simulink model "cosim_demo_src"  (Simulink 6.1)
settings: Solver=ode45  StartTime=0.0  StopTime=300  RelTol=1e-3
undefined symbols (not defined in the file or in its folder): netlist
libraries: xbsIndex_r3 x8

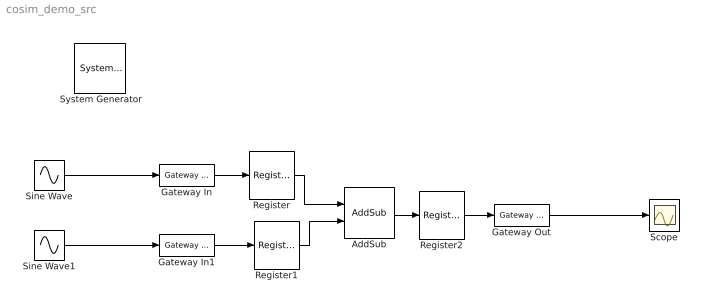
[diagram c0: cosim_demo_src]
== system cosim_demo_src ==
  " System Generator" : xbsIndex_r3/ System Generator  Tag=genX  xilinxfamily=Virtex2P  part=xc2vp70  speed=-5  package=ff1704  synthesis_tool=XST  directory=./netlist  testbench=off  simulink_period=1  sysclk_period=25  incr_netlist=off  trim_vbits=Everywhere in SubSystem  dbl_ovrd=According to Block Masks  core_generation=According to Block Masks  run_coregen=off  deprecated_control=off  eval_field=0
  AddSub : xbsIndex_r3/AddSub  mode=Addition  precision=Full  arith_type=Unsigned  n_bits=8  bin_pt=2  quantization=Truncate  overflow=Wrap  latency=0  explicit_period=off  period=1  use_carryin=off  use_carryout=off  en=off  dbl_ovrd=off  show_param=off  use_core=on  pipeline=off  use_rpm=off  gen_core=off
  Gateway In : xbsIndex_r3/Gateway In  arith_type="Signed  (2's comp)"  n_bits=12  bin_pt=0  quantization=Truncate  overflow=Wrap  period=1  timing_constraint=None  locs_specified=off  LOCs={}  needs_fixed_name=off  dbl_ovrd=off  show_param=off
  Gateway In1 : xbsIndex_r3/Gateway In  arith_type="Signed  (2's comp)"  n_bits=12  bin_pt=0  quantization=Truncate  overflow=Wrap  period=1  timing_constraint=None  locs_specified=off  LOCs={}  needs_fixed_name=off  dbl_ovrd=off  show_param=off
  Gateway Out : xbsIndex_r3/Gateway Out  output_type=Double  nbits=8  bin_pt=6  arith_type=Boolean  quantization=Truncate  overflow=Wrap  hdl_port=on  timing_constraint=None  locs_specified=off  LOCs={}  needs_fixed_name=off  show_param=off
  Register : xbsIndex_r3/Register  init=0  reg_only_valid=off  explicit_period=off  period=1  rst=off  en=off  out_en=off  dbl_ovrd=off  show_param=off
  Register1 : xbsIndex_r3/Register  init=0  reg_only_valid=off  explicit_period=off  period=1  rst=off  en=off  out_en=off  dbl_ovrd=off  show_param=off
  Register2 : xbsIndex_r3/Register  init=0  reg_only_valid=off  explicit_period=off  period=1  rst=off  en=off  out_en=off  dbl_ovrd=off  show_param=off
  Scope : Scope
  Sine Wave : Sin  Amplitude=2000  Frequency=.1  SampleTime=1
  Sine Wave1 : Sin  Amplitude=1000  Frequency=.3  SampleTime=1
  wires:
  Sine Wave/1 -> Gateway In/1
  Sine Wave1/1 -> Gateway In1/1
  Gateway In/1 -> Register/1
  Gateway In1/1 -> Register1/1
  Register/1 -> AddSub/1
  Register1/1 -> AddSub/2
  AddSub/1 -> Register2/1
  Register2/1 -> Gateway Out/1
  Gateway Out/1 -> Scope/1
